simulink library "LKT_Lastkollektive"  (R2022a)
settings: Solver=VariableStepAuto  StartTime=0.0  StopTime=10.0  RelTol=1e-3
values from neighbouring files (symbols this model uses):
  PAR_LKT_Deckenhoehe = 2.5    [parameter_LKT.m]
  PAR_LKT_Etagen = 2    [parameter_LKT.m]
  PAR_LKT_Fensterflaeche = 25    [parameter_LKT.m]
  PAR_LKT_Grundflaeche = 100    [parameter_LKT.m]
  PAR_LKT_OffSet = -20    [parameter_LKT.m]
  PAR_LKT_Strompreis = 0.3606    [parameter_LKT.m]
  PAR_LKT_StromverbrauchProPerson = 6.8    [parameter_LKT.m]
  PAR_LKT_Urlaubstag = 0    [parameter_LKT.m]
  PAR_LKT_WasserverbrauchProPerson = 0.1230    (= 0.123)    [parameter_LKT.m]
  PAR_LKT_Wochenendtag = 1    [parameter_LKT.m]
  PAR_LKT_zweiErwachsene = 2    [parameter_LKT.m]
  PAR_LKT_zweiKinder = 2    [parameter_LKT.m]
undefined symbols (not defined in the file or in its folder): PAR_LKT_Temperatur

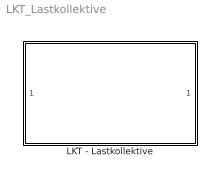
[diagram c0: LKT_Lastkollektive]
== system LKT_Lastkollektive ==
  LKT - Lastkollektive : Subsystem

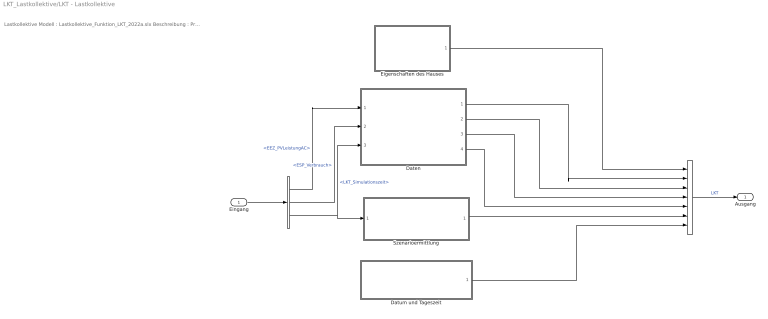
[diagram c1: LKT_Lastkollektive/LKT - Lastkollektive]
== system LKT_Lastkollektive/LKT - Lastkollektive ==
  note: Lastkollektive Modell : Lastkollektive_Funktion_LKT_2022a.slx Beschreibung : Programm für die Lastkollektive im SoSe 2023 SDE im Simulationsprojekt Einfamilienhaus Implementierung : Simulink (R2022a) Toolbox : Autor : Schartner, David & Stute, Marvin Bemerkung :
  Eingang : Inport
  " " : BusSelector  OutputSignals=EEZ_PVLeistungAC,ESP_Verbrauch,LKT.LKT_Simulationszeit
  "  " : BusCreator  Inputs=7
  Daten : Subsystem
  Datum und Tageszeit : Subsystem
  Eigenschaften des Hauses : Subsystem
  Szenarioermittlung : Subsystem
  Ausgang : Outport
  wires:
  Eigenschaften des Hauses/1(LKT_Eigenschaften_des_Hauses) -> "  "/1
  Daten/1(LKT_Temperatur) -> "  "/2
  "  "/1 -> Ausgang/1  "LKT"
  Eingang/1 -> " "/1
  Daten/2(LKT_Stromkosten) -> "  "/3
  Daten/3(LKT_Wasserverbrauch) -> "  "/4
  Datum und Tageszeit/1(LKT_Simulationszeit) -> "  "/7
  Szenarioermittlung/1(LKT_PersonenZuhause) -> "  "/6
  " "/3 -> Daten/3(LKT_Simulationszeit), Szenarioermittlung/1(LKT_Simulationszeit)  "<LKT_Simulationszeit>"
  " "/2 -> Daten/2(ESP_Verbrauch)  "<ESP_Verbrauch>"
  " "/1 -> Daten/1(EEZ_PVLeistungAC)  "<EEZ_PVLeistungAC>"
  Daten/4(LKT_Stromverbrauch) -> "  "/5

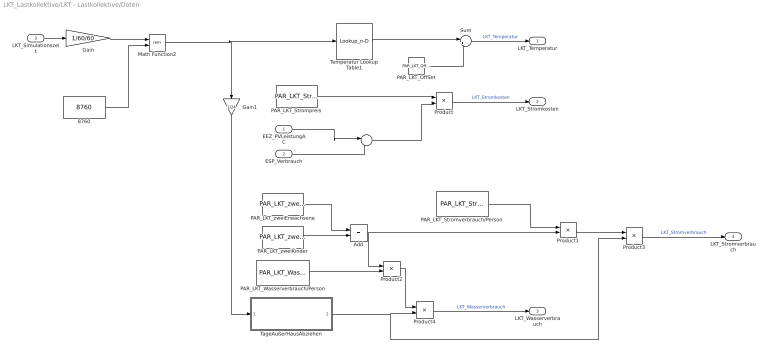
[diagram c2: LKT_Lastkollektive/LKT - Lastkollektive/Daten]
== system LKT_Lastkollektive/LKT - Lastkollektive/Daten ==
  EEZ_PVLeistungAC : Inport
  ESP_Verbrauch : Inport  Port=2
  LKT_Simulationszeit : Inport  Port=3
  " " : Sum  Inputs=|-+
  8760 : Constant  Value=8760
  Add : Sum
  Gain : Gain  Gain=1/60/60
  Gain1 : Gain  Gain=1/24
  Math Function2 : Math  Operator=rem
  PAR_LKT_OffSet : Constant  Value=PAR_LKT_OffSet
  PAR_LKT_Strompreis : Constant  Value=PAR_LKT_Strompreis
  PAR_LKT_Stromverbrauch/Person : Constant  Value=PAR_LKT_StromverbrauchProPerson
  PAR_LKT_Wasserverbrauch/Person : Constant  Value=PAR_LKT_WasserverbrauchProPerson
  PAR_LKT_zweiErwachsene : Constant  Value=PAR_LKT_zweiErwachsene
  PAR_LKT_zweiKinder : Constant  Value=PAR_LKT_zweiKinder
  Product{,1..4} (5 alike) : Product
  Sum : Sum  Inputs=|++
  TageAußerHausAbziehen : MATLAB Function  TreatAsAtomicUnit=on  SystemSampleTime=10
  Temperatur Lookup Table1 : Lookup_n-D  NumberOfTableDimensions=1  BreakpointsForDimension1=1:8760  Table=PAR_LKT_Temperatur  InternalRulePriority=Speed  RndMeth=Simplest
  LKT_Temperatur : Outport
  LKT_Stromkosten : Outport  Port=2
  LKT_Wasserverbrauch : Outport  Port=3
  LKT_Stromverbrauch : Outport  Port=4
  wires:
  PAR_LKT_Strompreis/1 -> Product/1
  ESP_Verbrauch/1 -> " "/2
  Product/1 -> LKT_Stromkosten/1  "LKT_Stromkosten"
  EEZ_PVLeistungAC/1 -> " "/1
  " "/1 -> Product/2
  Product4/1 -> LKT_Wasserverbrauch/1  "LKT_Wasserverbrauch"
  PAR_LKT_Wasserverbrauch/Person/1 -> Product2/2
  TageAußerHausAbziehen/1(TageZuhause) -> Product3/2, Product4/2
  LKT_Simulationszeit/1 -> Gain/1
  Gain1/1 -> TageAußerHausAbziehen/1(aktuellerTag)
  PAR_LKT_zweiErwachsene/1 -> Add/1
  Add/1 -> Product1/2, Product2/1
  PAR_LKT_zweiKinder/1 -> Add/2
  Product2/1 -> Product4/1
  PAR_LKT_Stromverbrauch/Person/1 -> Product1/1
  Product1/1 -> Product3/1
  Product3/1 -> LKT_Stromverbrauch/1  "LKT_Stromverbrauch"
  Gain/1 -> Math Function2/1
  8760/1 -> Math Function2/2
  Math Function2/1 -> Temperatur Lookup Table1/1, Gain1/1
  Temperatur Lookup Table1/1 -> Sum/1
  PAR_LKT_OffSet/1 -> Sum/2
  Sum/1 -> LKT_Temperatur/1  "LKT_Temperatur"

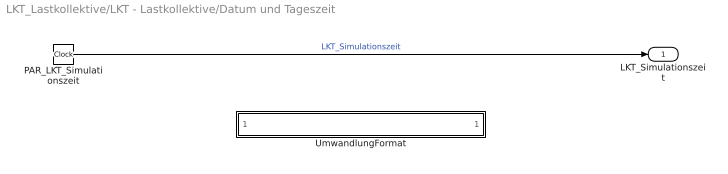
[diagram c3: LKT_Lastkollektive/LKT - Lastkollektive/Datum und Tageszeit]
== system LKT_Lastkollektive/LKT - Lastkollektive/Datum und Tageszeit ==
  PAR_LKT_Simulationszeit : Clock
  UmwandlungFormat : MATLAB Function  Commented=on  TreatAsAtomicUnit=on
  LKT_Simulationszeit : Outport
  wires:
  PAR_LKT_Simulationszeit/1 -> LKT_Simulationszeit/1  "LKT_Simulationszeit"

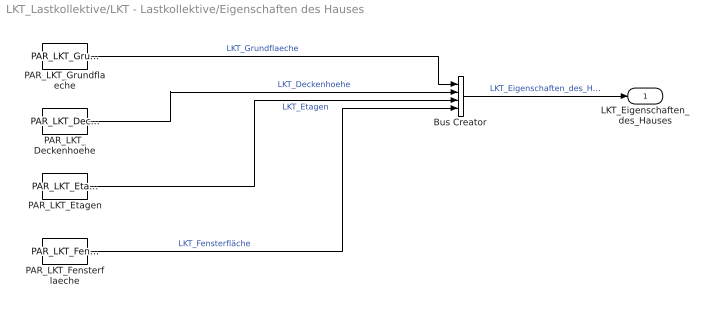
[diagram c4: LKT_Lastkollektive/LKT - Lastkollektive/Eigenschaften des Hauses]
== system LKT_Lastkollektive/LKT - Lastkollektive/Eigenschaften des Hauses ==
  Bus Creator : BusCreator  Inputs=4
  PAR_LKT_Deckenhoehe : Constant  Value=PAR_LKT_Deckenhoehe
  PAR_LKT_Etagen : Constant  Value=PAR_LKT_Etagen
  PAR_LKT_Fensterflaeche : Constant  Value=PAR_LKT_Fensterflaeche
  PAR_LKT_Grundflaeche : Constant  Value=PAR_LKT_Grundflaeche
  LKT_Eigenschaften_des_Hauses : Outport
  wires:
  PAR_LKT_Grundflaeche/1 -> Bus Creator/1  "LKT_Grundflaeche"
  PAR_LKT_Deckenhoehe/1 -> Bus Creator/2  "LKT_Deckenhoehe"
  PAR_LKT_Etagen/1 -> Bus Creator/3  "LKT_Etagen"
  PAR_LKT_Fensterflaeche/1 -> Bus Creator/4  "LKT_Fensterfläche"
  Bus Creator/1 -> LKT_Eigenschaften_des_Hauses/1  "LKT_Eigenschaften_des_Hauses"

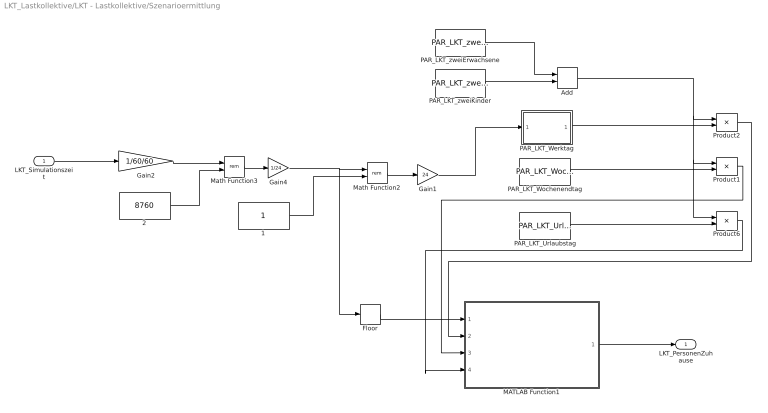
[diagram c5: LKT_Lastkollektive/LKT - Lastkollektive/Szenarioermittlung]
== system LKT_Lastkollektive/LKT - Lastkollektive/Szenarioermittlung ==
  LKT_Simulationszeit : Inport
  1 : Constant
  2 : Constant  Value=8760
  Add : Sum
  Floor : Rounding
  Gain1 : Gain  Gain=24
  Gain2 : Gain  Gain=1/60/60
  Gain4 : Gain  Gain=1/24
  MATLAB Function1 : MATLAB Function  TreatAsAtomicUnit=on
  Math Function2 : Math  Operator=rem
  Math Function3 : Math  Operator=rem
  PAR_LKT_Urlaubstag : Constant  Value=PAR_LKT_Urlaubstag
  PAR_LKT_Werktag : MATLAB Function  TreatAsAtomicUnit=on
  PAR_LKT_Wochenendtag : Constant  Value=PAR_LKT_Wochenendtag
  PAR_LKT_zweiErwachsene : Constant  Value=PAR_LKT_zweiErwachsene
  PAR_LKT_zweiKinder : Constant  Value=PAR_LKT_zweiKinder
  Product1 : Product
  Product2 : Product
  Product6 : Product
  LKT_PersonenZuhause : Outport
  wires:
  PAR_LKT_zweiErwachsene/1 -> Add/1
  PAR_LKT_zweiKinder/1 -> Add/2
  Gain4/1 -> Floor/1, Math Function2/1
  PAR_LKT_Urlaubstag/1 -> Product6/2
  Floor/1 -> MATLAB Function1/1(aktuellerTag)
  PAR_LKT_Wochenendtag/1 -> Product1/2
  Gain1/1 -> PAR_LKT_Werktag/1(u)
  Product6/1 -> MATLAB Function1/4(UrlaubstagP)
  LKT_Simulationszeit/1 -> Gain2/1
  Add/1 -> Product6/1, Product1/1, Product2/1
  MATLAB Function1/1(LKT_PersonenZuhause) -> LKT_PersonenZuhause/1
  Math Function2/1 -> Gain1/1
  1/1 -> Math Function2/2
  Product1/1 -> MATLAB Function1/3(WochenendTagP)
  PAR_LKT_Werktag/1(y) -> Product2/2
  Product2/1 -> MATLAB Function1/2(WochentagP)
  Gain2/1 -> Math Function3/1
  2/1 -> Math Function3/2
  Math Function3/1 -> Gain4/1

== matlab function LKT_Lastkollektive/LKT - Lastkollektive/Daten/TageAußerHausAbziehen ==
function TageZuhause = fcn(aktuellerTag)

% Die Funktion zieht die Tage von dem Tageszähler ab, an denen die Familie
% außer Haus ist über den Sommer- bzw. Winterurlaub

persistent TageAusserHausSommer TageAusserHausWinter ersterDurchlauf Sommerurlaub Winterurlaub

if isempty(ersterDurchlauf)

    Sommerurlaub = [213 227]; 
    Winterurlaub = [358 365]; 
    TageAusserHausSommer = 0; % initialisiert den Zähler für Tage die Sie nicht zuhause sind
    TageAusserHausWinter = 0;
    ersterDurchlauf = 1;
end

if aktuellerTag>=Sommerurlaub(1) && aktuellerTag <= Sommerurlaub(2)
    
    TageAusserHausSommer = aktuellerTag - Sommerurlaub(1);
    
end

if aktuellerTag>=Winterurlaub(1) && aktuellerTag <= Winterurlaub(2)

    TageAusserHausWinter = aktuellerTag - Winterurlaub(1);

end

TageZuhause = aktuellerTag - TageAusserHausSommer - TageAusserHausWinter;

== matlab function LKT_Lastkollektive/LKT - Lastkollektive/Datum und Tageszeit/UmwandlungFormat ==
function LKT_aktuellesDatum = fcn(PAR_LKT_Simulationszeit)

startDatum = datetime(2022, 1, 1); % Startet die Daumsermittlung beim Datum 1.1.2022
simuliertesDatum = startDatum + seconds(PAR_LKT_Simulationszeit); % addiert die Simulationszeit auf StartDatum

[Jahr, Monat, Tag, Stunde, Minute, Sekunde] = datevec(simuliertesDatum);


LKT_aktuellesDatum = round([Jahr Monat Tag Stunde Minute Sekunde]); % Bringt die einzelnen Werte in richtige Form für Output
end

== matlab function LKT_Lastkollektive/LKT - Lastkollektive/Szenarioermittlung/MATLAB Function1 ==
function LKT_PersonenZuhause = fcn(aktuellerTag, WochentagP, WochenendTagP, UrlaubstagP)


LKT_PersonenZuhause = 0; % Initialisiert die Ausgangsvariable
Sommerurlaub = [213 227]; % Tage in denen die Familie im Sommerurlaub ist
Winterurlaub = [358 365]; % Tage in denen die Faimilie im Winterurlaub ist

if aktuellerTag>=Sommerurlaub(1) && aktuellerTag <= Sommerurlaub(2) || aktuellerTag>=Winterurlaub(1) && aktuellerTag <= Winterurlaub(2)
    % Überprüft ob sich die Personen im Urlaub befinden und wählt falls es
    % der Fall ist das passende Szenario aus
    LKT_PersonenZuhause = UrlaubstagP;
    return
end

day  = mod(aktuellerTag, 7); % Der Rest aus der Division mit 7 gibt an, welcher Wochentag aktuell ist (Zahl zwischen 0 - 6)

if day == 5 || day == 6 % Die Tage 5 & 6 sind Samstag und Sonntag, also Wochenende
    weekend = true;
else
    weekend = false;
end

% Überprüft ob Wochenende ist und wählt das passende Szenario aus
if weekend == false
    LKT_PersonenZuhause = WochentagP;
    return
elseif weekend == true
    LKT_PersonenZuhause = WochenendTagP;
    return
end

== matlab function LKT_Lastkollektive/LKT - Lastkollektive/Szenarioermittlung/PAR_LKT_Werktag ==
function y = fcn(u)

if u >= 0 && u < 8
    y = 1;
elseif u >= 8 && u < 14
    y = 0;
elseif u >= 14 && u < 18
    y = 0.75;
else
    y = 1;
end
